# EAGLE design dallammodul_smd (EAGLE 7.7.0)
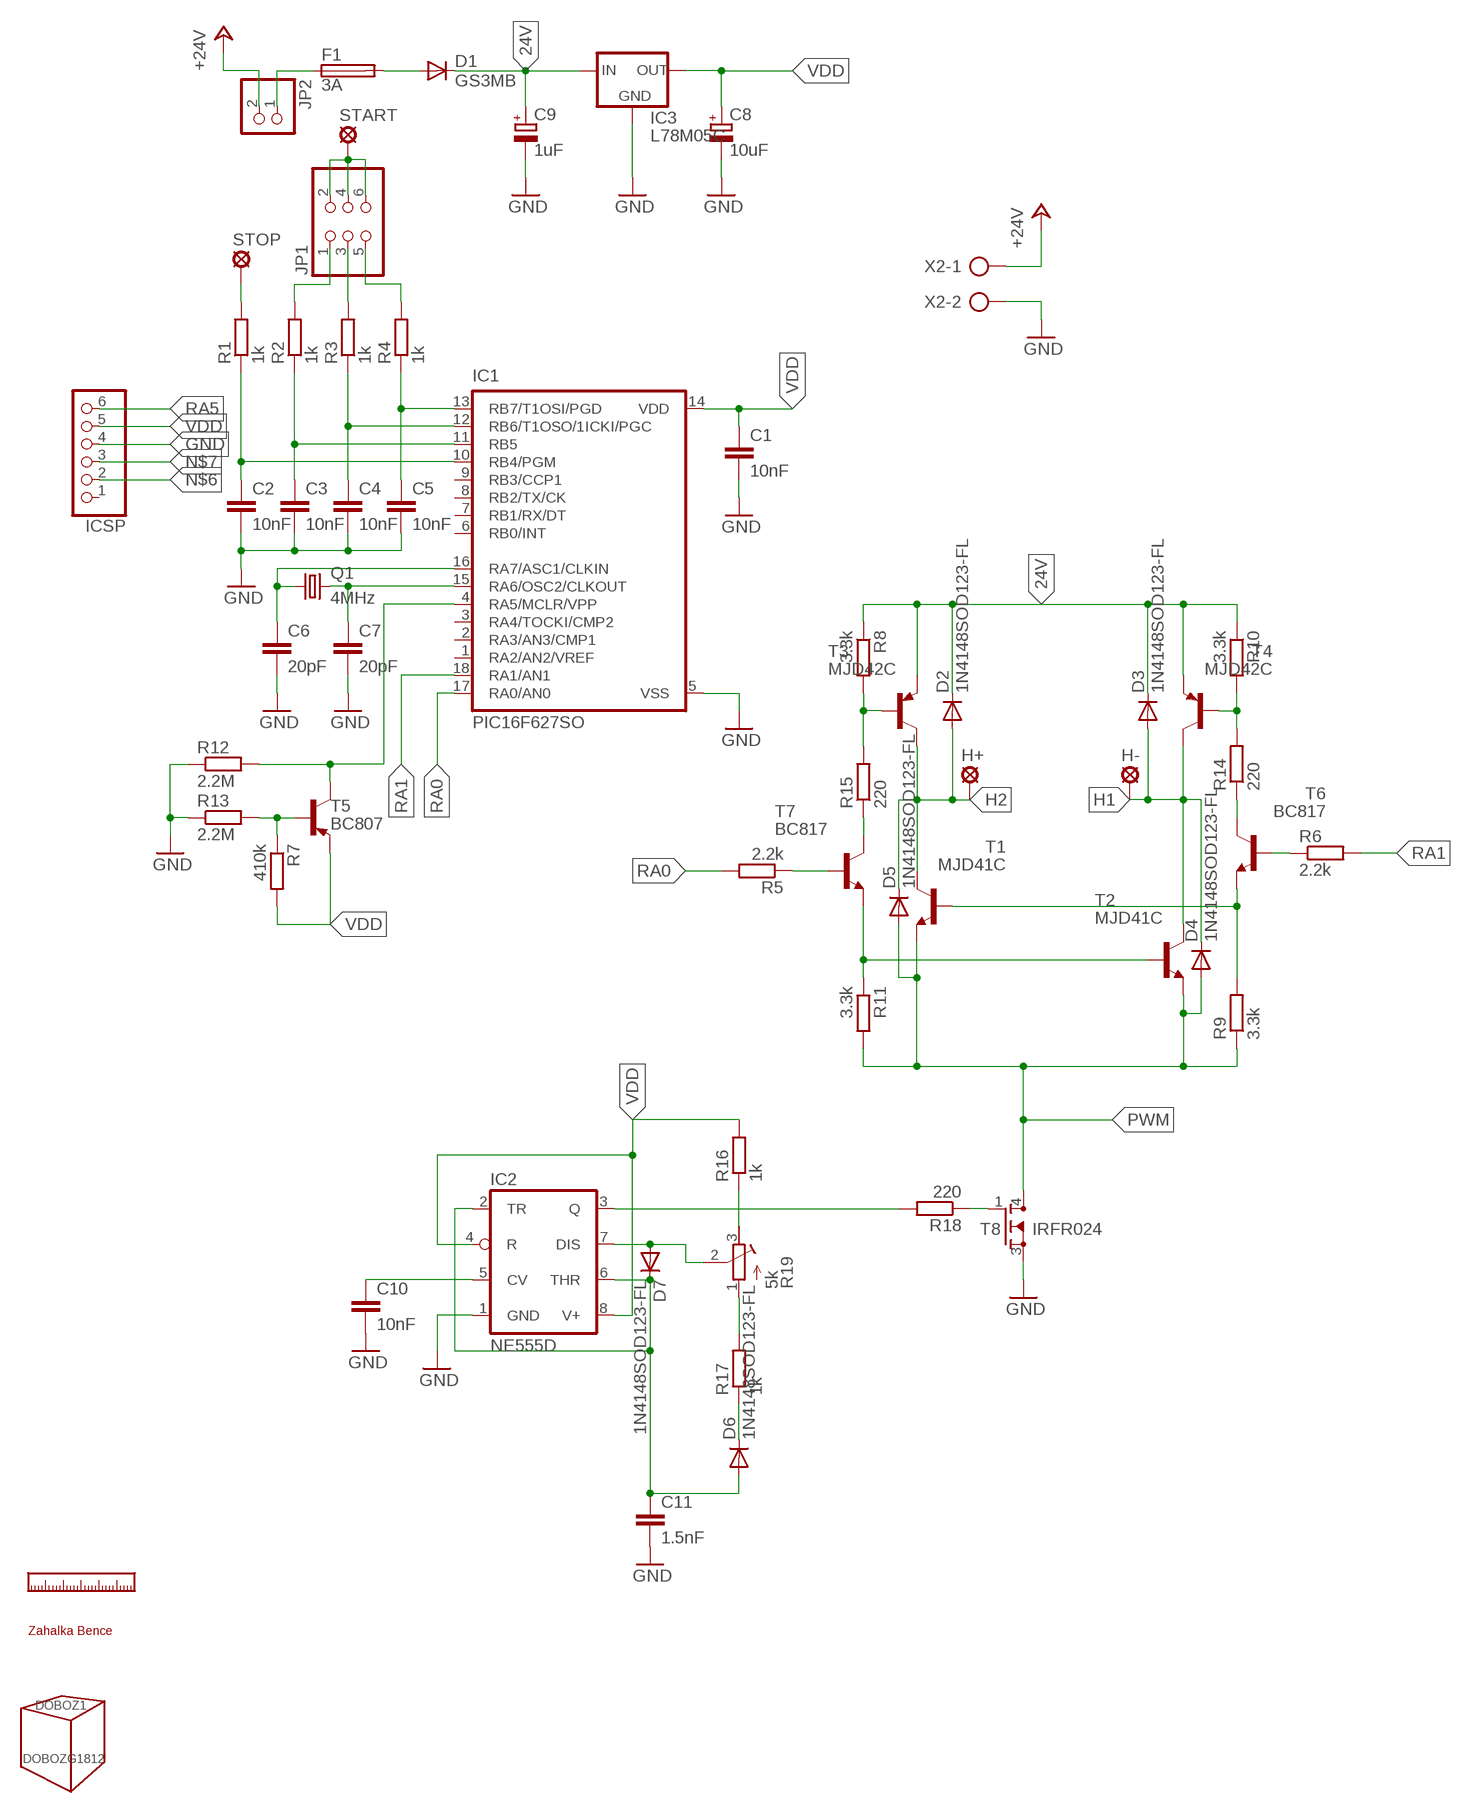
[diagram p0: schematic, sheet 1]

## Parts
C1  10nF  C-EUC0805  [C0805]
C2  10nF  C-EUC0805  [C0805]
C3  10nF  C-EUC0805  [C0805]
C4  10nF  C-EUC0805  [C0805]
C5  10nF  C-EUC0805  [C0805]
C6  20pF  C-EUC0805  [C0805]
C7  20pF  C-EUC0805  [C0805]
C8  10uF  CPOL-EU153CLV-0505  [153CLV-0505]
C9  1uF  CPOL-EU153CLV-0405  [153CLV-0405]
C10  10nF  C-EUC0805  [C0805]
C11  1.5nF  C-EUC0805  [C0805]
D1  GS3MB  DIODE-DO214AA  [DO214AA]
D2  1N4148SOD123-FL  [SOD123FL]
D3  1N4148SOD123-FL  [SOD123FL]
D4  1N4148SOD123-FL  [SOD123FL]
D5  1N4148SOD123-FL  [SOD123FL]
D6  1N4148SOD123-FL  [SOD123FL]
D7  1N4148SOD123-FL  [SOD123FL]
DOBOZ1  DOBOZG1812  [G1812]
F1  3A  BIZTOSITEK  [OMNIBLOK]
H+  LSP10  [LSP10]
H-  LSP10  [LSP10]
IC1  PIC16F627SO  [SO-18W]
IC2  NE555D  [SO08]
IC3  L78M05C  L78MXXCDPAK  [TO252]
ICSP  PINHD-1X6  [1X06]
JP1  PINHD-2X3  [2X03]
JP2  PINHD-1X2  [1X02]
Q1  4MHz  CRYSTALHC49UP  [HC49UP]
R1  1k  R-EU_R0805  [R0805]
R2  1k  R-EU_R0805  [R0805]
R3  1k  R-EU_R0805  [R0805]
R4  1k  R-EU_R0805  [R0805]
R5  2.2k  R-EU_R0805  [R0805]
R6  2.2k  R-EU_R0805  [R0805]
R7  410k  R-EU_R0805  [R0805]
R8  3.3k  R-EU_R0805  [R0805]
R9  3.3k  R-EU_R0805  [R0805]
R10  3.3k  R-EU_R0805  [R0805]
R11  3.3k  R-EU_R0805  [R0805]
R12  2.2M  R-EU_R0805  [R0805]
R13  2.2M  R-EU_R0805  [R0805]
R14  220  R-EU_R0805  [R0805]
R15  220  R-EU_R0805  [R0805]
R16  1k  R-EU_R0805  [R0805]
R17  1k  R-EU_R0805  [R0805]
R18  220  R-EU_R0805  [R0805]
R19  5k  R-TRIMM64W  [RTRIM64W]
START  LSP10  [LSP10]
STOP  LSP10  [LSP10]
T1  MJD41C  TRANSISTOR-NPNDPAK  [TO252]
T2  MJD41C  TRANSISTOR-NPNDPAK  [TO252]
T3  MJD42C  TRANSISTOR-PNPDPAK  [TO252]
T4  MJD42C  TRANSISTOR-PNPDPAK  [TO252]
T5  BC807  TRANSISTOR-PNPSOT23-BEC  [SOT23]
T6  BC817  TRANSISTOR-NPNSOT23-BEC  [SOT23]
T7  BC817  TRANSISTOR-NPNSOT23-BEC  [SOT23]
T8  IRFR024  NPN-FETDPAK  [TO252]
U$1  VONALZO  [VONALZO]
X2  AK300/2  [AK300/2]
ZB1  ZB  [ZB]

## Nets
24V: C9.+ D1.C D2.C D3.C IC3.1(IN) R8.1 R10.1 T3.3(E) T4.3(E)
+24V: JP2.2 X2.1
GND: C1.2 C2.2 C3.2 C4.2 C5.2 C6.2 C7.2 C8.- C9.- C10.2 C11.2 IC1.5(VSS) IC2.1(GND) IC3.4(GND) ICSP.4 R12.1 R13.1 T8.3(S) X2.2
H1: D3.A D4.C H-.MP T2.4(C) T4.4(C)
H2: D2.A D5.C H+.MP T1.4(C) T3.4(C)
N$1: C6.1 IC1.16(RA7/ASC1/CLKIN) Q1.1
N$2: C7.1 IC1.15(RA6/OSC2/CLKOUT) Q1.2
N$3: C2.1 IC1.10(RB4/PGM) R1.1
N$4: C3.1 IC1.11(RB5) R2.1
N$5: R5.1 T7.1(B)
N$6: C4.1 IC1.12(RB6/T1OSO/1ICKI/PGC) ICSP.2 R3.1
N$7: C5.1 IC1.13(RB7/T1OSI/PGD) ICSP.3 R4.1
N$8: JP1.5 R4.2
N$9: JP1.3 R3.2
N$10: JP1.1 R2.2
N$11: R1.2 STOP.MP
N$12: R16.1 R19.3(A)
N$13: R17.2 R19.1(E)
N$14: D1.A F1.2
N$15: R8.2 R15.2 T3.1(B)
N$16: R10.2 R14.2 T4.1(B)
N$17: R7.1 R13.2 T5.1(B)
N$18: R15.1 T7.3(C)
N$19: R6.1 T6.1(B)
N$20: R11.1 T2.1(B) T7.2(E)
N$21: IC2.3(Q) R18.2
N$22: R9.2 T1.1(B) T6.2(E)
N$23: R14.1 T6.3(C)
N$24: R18.1 T8.1(G)
N$25: JP1.2 JP1.4 JP1.6 START.MP
N$26: D7.A IC2.7(DIS) R19.2(S)
N$27: D6.C R17.1
N$28: C11.1 D6.A D7.C IC2.2(TR) IC2.6(THR)
N$30: C10.1 IC2.5(CV)
N$31: F1.1 JP2.1
PWM: D4.A D5.A R9.1 R11.2 T1.3(E) T2.3(E) T8.4(D)
RA0: IC1.17(RA0/AN0) R5.2
RA1: IC1.18(RA1/AN1) R6.2
RA5: IC1.4(RA5/MCLR/VPP) ICSP.6 R12.2 T5.3(C)
VDD: C1.1 C8.+ IC1.14(VDD) IC2.4(R) IC2.8(V+) IC3.3(OUT) ICSP.5 R7.2 R16.2 T5.2(E)
Unconnected: IC1.1(RA2/AN2/VREF) IC1.2(RA3/AN3/CMP1) IC1.3(RA4/TOCKI/CMP2) IC1.6(RB0/INT) IC1.7(RB1/RX/DT) IC1.8(RB2/TX/CK) IC1.9(RB3/CCP1) ICSP.1

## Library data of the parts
C1-C7 C10 C11 = rcl:C-EU: CAPACITOR, European symbol
C8 C9 = rcl:CPOL-EU: POLARIZED CAPACITOR, European symbol
D1 = diode:DIODE-: DIODE
D2-D7 = diode:1N4148: DIODE
DOBOZ1 = sajat:DOBOZ: Ha eleve dobozba tervezném az áramkört, akkor miért ne legyen meg alkatrészként?
F1 = sajat:BIZTOSITEK
H+ H- START STOP = sajat:LSP10: SOLDER PAD
IC1 = microchip:PIC16*F62: FLASH-Based 8-Bit CMOS Microcontroller Source: http://ww1.microchip.com/downloads/en/DeviceDoc/40300C.pdf; MF: MICROCHIP; MPN: PIC16F627-04/SO; OC_FARNELL: 1084265; OC_NEWARK: 69K7632
IC2 = linear:*555: TIMER
IC3 = sajat:L78MXXC
ICSP = pinhead:PINHD-1X6: PIN HEADER
JP1 = pinhead:PINHD-2X3: PIN HEADER
JP2 = pinhead:PINHD-1X2: PIN HEADER
Q1 = crystal:CRYSTAL: CRYSTAL; OC_FARNELL: unknown; OC_NEWARK: unknown
R1-R18 = rcl:R-EU_: RESISTOR, European symbol
R19 = resistor:R-TRIMM: Trimm resistor
T1 T2 T6 T7 = sajat:TRANSISTOR-NPN
T3-T5 = sajat:TRANSISTOR-PNP
T8 = sajat:NPN-FET: NPN FET
U$1 = sajat:VONALZO: vonalzó
X2 = con-ptr500:AK300/2: CONNECTOR; OC_FARNELL: unknown; OC_NEWARK: unknown
ZB1 = sajat:ZB: Zahalka Bence monogram

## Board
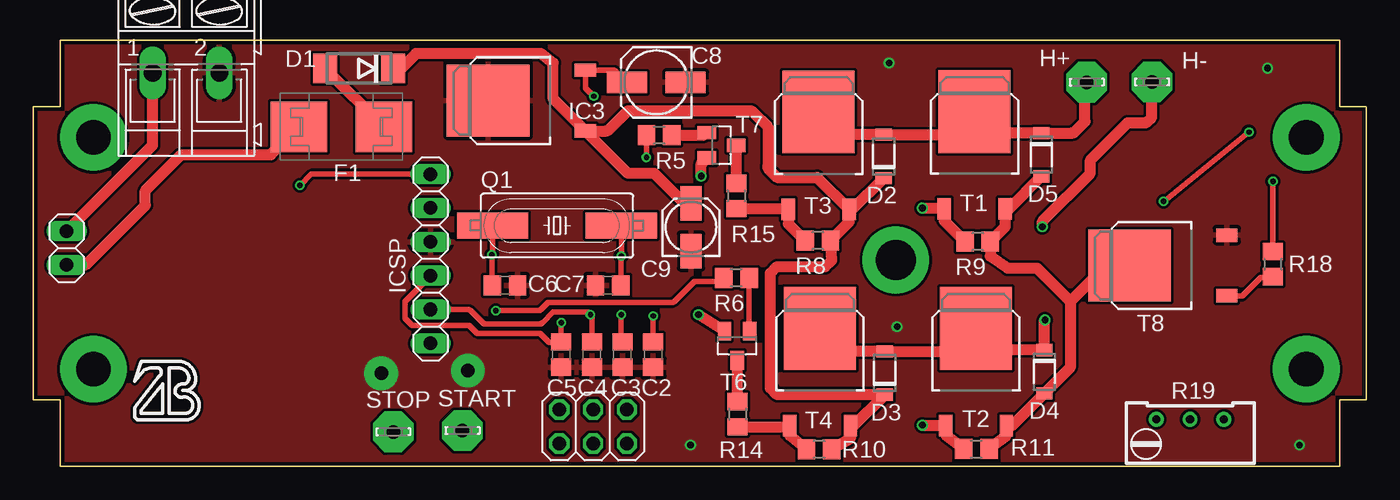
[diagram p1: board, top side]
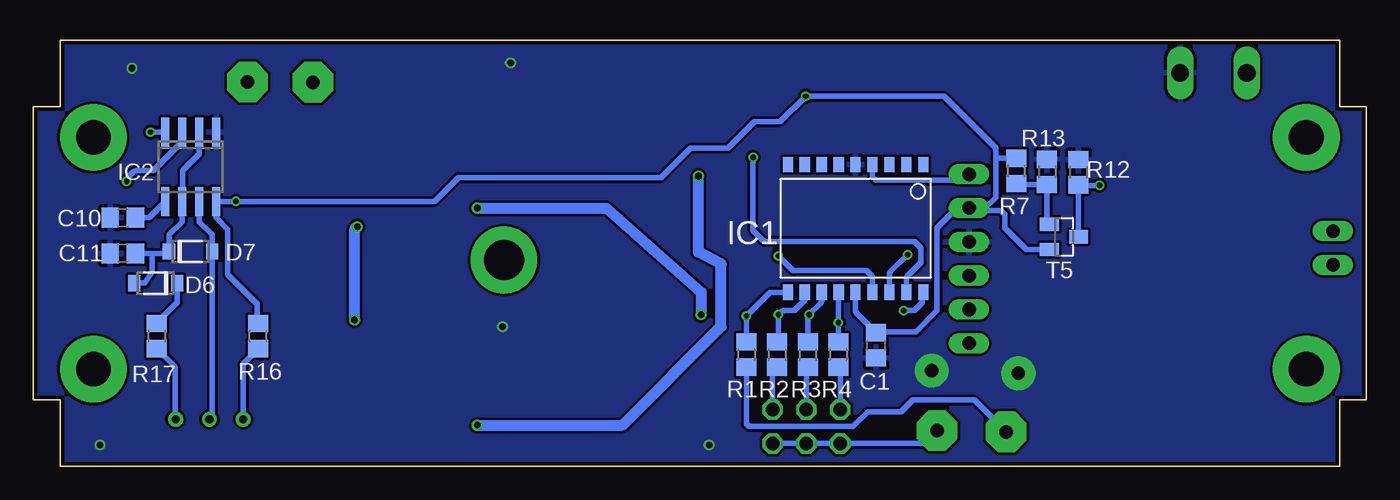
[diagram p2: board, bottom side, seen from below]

Size 100 x 32 mm. Coordinates in mm from the lower left corner, seen from the top.
Copper layers (1*16): Top 0.035mm / dielectric 1.5mm / Bottom 0.035mm
Design rules "dirt_cheap_dirty_boards.v1": minimum track width 5mil, minimum drill 12mil, track to track 5mil, track to pad 5mil, pad to pad 5mil, via to via 5mil, smd to smd 0mil, copper to edge 10mil, drill to drill 10mil, minimum pad ring 10mil, minimum via ring 6mil, stop-mask expansion 2mil, vias tented up to drill 25mil, thermal gap 10mil

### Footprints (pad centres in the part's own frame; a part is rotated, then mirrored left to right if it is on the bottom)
C0805 = smd 1.3 x 1.5: 1 -0.95,0; 2 0.95,0
153CLV-0505 = smd 3 x 1.6: + 2.2,0; - -2.2,0
153CLV-0405 = smd 2.6 x 1.6: + 1.8,0; - -1.8,0
DO214AA = smd 1.8 x 2.2: A 2.55,0; C -2.55,0
SOD123FL = smd 0.91 x 1.22: A 1.625,0; C -1.625,0
G1812 = drill 2.6 pad 5: P$1 -45.5,-8.7; P$2 45.5,-8.7; P$3 45.5,8.7; P$4 -45.5,8.7
OMNIBLOK = smd 4.24 x 3.81: 1 -3.185,0; 2 3.185,0
LSP10 = drill 1.016 pad 3.048 octagon: MP 0,0
SO-18W = smd 0.762 x 1.143: 1 -5.08,-4.788; 2 -3.81,-4.788; 3 -2.54,-4.788; 4 -1.27,-4.788; 5 0,-4.788; 6 1.27,-4.788; 7 2.54,-4.788; 8 3.81,-4.788; 9 5.08,-4.788; 10 5.08,4.788; 11 3.81,4.788; 12 2.54,4.788; 13 1.27,4.788; 14 0,4.788; 15 -1.27,4.788; 16 -2.54,4.788; 17 -3.81,4.788; 18 -5.08,4.788
SO08 = smd 0.6 x 2.2: 1 -1.905,-2.6; 2 -0.635,-2.6; 3 0.635,-2.6; 4 1.905,-2.6; 5 1.905,2.6; 6 0.635,2.6; 7 -0.635,2.6; 8 -1.905,2.6
TO252 = smd 1 x 1.6: 1 -2.28,-4.8; 3 2.28,-4.8 | smd 5.4 x 6.2: 4 0,2.5
1X06 = drill 1.016 long: 1 -6.35,0; 2 -3.81,0; 3 -1.27,0; 4 1.27,0; 5 3.81,0; 6 6.35,0
2X03 = drill 1.016 octagon: 1 -2.54,-1.27; 2 -2.54,1.27; 3 0,-1.27; 4 0,1.27; 5 2.54,-1.27; 6 2.54,1.27
1X02 = drill 1.016 long: 1 -1.27,0; 2 1.27,0
HC49UP = smd 5.334 x 1.93: 1 -4.826,0; 2 4.826,0
R0805 = smd 1.3 x 1.5: 1 -0.95,0; 2 0.95,0
RTRIM64W = drill 0.61: 1 1.27,-2.54; 2 1.27,0; 3 1.27,2.54
SOT23 = smd 1 x 1.4: 1 -0.95,-1.1; 2 0.95,-1.1; 3 0,1.1
AK300/2 = drill 1.321 long: 1 -2.515,0; 2 2.489,0

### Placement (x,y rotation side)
C1  36.78,9.1 270 bottom
C2  46.5,8.4 270 top
C3  44.2,8.4 270 top
C4  41.9,8.4 270 top
C5  39.6,8.4 270 top
C6  35.38,13.6 0 top
C7  43.13,13.6 180 top
C8  46.74,28.84 180 top
C9  49.34,17.97 90 top
C10  93.28,18.68 180 bottom
C11  93.28,16 180 bottom
D1  24.46,29.88 180 top
D2  63.8,23.28 90 top
D3  63.88,7.02 90 top
D4  75.85,7.11 270 top
D5  75.63,23.41 270 top
D6  90.82,13.76 180 bottom
D7  88.2,16.14 0 bottom
DOBOZ1  50,16 0 top
F1  23.1,25.5 0 top
H+  79.03,28.85 0 top
H-  83.93,28.87 0 top
IC1  38.31,17.87 180 bottom
IC2  88.2,22.49 180 bottom
IC3  36.62,27.47 90 top
ICSP  29.8,15.6 90 top
JP1  42,3 180 top
JP2  2.5,16.4 90 top
Q1  39.29,18.09 0 top
R1  46.5,8.4 270 bottom
R2  44.2,8.4 270 bottom
R3  41.9,8.4 270 bottom
R4  39.6,8.4 270 bottom
R5  46.95,24.86 180 top
R6  52.75,14.16 180 top
R7  26.24,22.19 90 bottom
R8  58.85,16.96 180 top
R9  70.85,16.88 180 top
R10  58.95,1.28 180 top
R11  70.75,1.32 0 top
R12  21.59,22.09 270 bottom
R13  23.94,22.11 270 bottom
R14  52.84,3.93 270 top
R15  52.74,20.31 270 top
R16  83.12,9.79 90 bottom
R17  90.74,9.79 270 bottom
R18  93.01,15.19 90 top
R19  86.79,2.27 90 top
START  32.2,2.7 0 top
STOP  27,2.6 0 top
T1  70.62,24.14 0 top
T2  70.72,7.86 0 top
T3  58.92,24.11 0 top
T4  59.02,7.86 0 top
T5  22.67,17.24 270 bottom
T6  52.8,9.07 180 top
T7  51.63,24.12 270 top
T8  84.74,15.09 90 top
U$1  not placed on the board
X2  11.47,29.55 0 top
ZB1  9.9,5.8 0 top

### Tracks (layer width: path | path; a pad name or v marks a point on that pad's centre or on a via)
24V
  Top 0.813: T3.3 61.2,18.36 R8.1 59.9,15.5 59.4,15 55.8,15 55.3,14.5 55.3,5.9 55.8,5.39 D3.C 61.55,3.06 T4.3 61.3,2.08 R10.1 | T3.3 61.45,19.31 D2.C | T3.3 58.81,21.7 55.8,21.7 55.19,22.31 arc-45 55.1,22.53 55.1,25.5 53.99,26.61 arc45 53.77,26.7 44.6,26.7 43.18,25.28 arc-45 42.96,25.19 IC3.1 | C9.+ 48.96,19.77 arc-45 48.74,19.86 46.6,22 44.74,22 arc-45 44.52,22.09 IC3.1 | IC3.1 39,27.6 39,30.28 38.08,31 28.7,31 27.58,29.88 D1.C
+24V
  Top 0.813: JP2.2 8.96,24.13 X2.1
GND  (via drill 0.5, 1 pad 2.54)
  other vias: 64.2,30.3 92.6,29.9 95,1.6 49.3,1.6 32.6,7.2 26.1,7 64.8,10.5
  pour Bottom (isolate 0.2): 2,32 98,32 98,27 100,27 100,5 98,5 98,0 2,0 2,5 0,5 0,27 2,27
  pour Top (isolate 0.2): 0,32.2 100.1,32.2 100.1,-1.3 0,-1.3 0,30.2
H1  (via drill 0.5)
  Top 0.813: T4.4 60.73,8.64 D3.A 69,8.64 T2.4 72.34,8.73 D4.C 75.85,10.88 arc-45 v75.9,11 | v75.7,18 75.7,18.27 arc-45 75.79,18.49 79.3,22 79.3,22.87 arc-45 79.39,23.09 82.1,25.8 83.37,25.8 arc45 83.59,25.89 83.9,26.2 83.9,28.8 arc-45 H-.MP
  Bottom 0.813: v75.9,11 75.9,17.67 arc45 75.81,17.89 v75.7,18
H2
  Top 0.813: 70.98,26.28 72.22,25.04 D5.C 77.9,25.04 arc45 78.13,25.13 78.9,25.9 78.9,28.59 arc-45 78.99,28.81 H+.MP | 70.98,26.28 T1.4 | T3.4 60.62,24.9 D2.A 69.61,24.9 70.98,26.28
HUTOBORDA  (via drill 3 pad 5)
  other vias: 64.7,15.5
N$1  (via drill 0.4)
  Top 0.406: Q1.1 34.46,16.05 arc-45 v34.4,15.9 arc-45 34.43,15.83 C6.1
  Bottom 0.406: IC1.16 35.77,14.4 arc45 35.68,14.62 v34.4,15.9
N$2  (via drill 0.4)
  Top 0.406: Q1.2 44.12,15.84 arc-45 v44.1,15.8 arc45 44.08,15.75 C7.1
  Bottom 0.406: IC1.15 37.04,14.11 arc-45 37.13,14.33 37.5,14.7 42.87,14.7 arc45 43.09,14.79 v44.1,15.8
N$3  (via drill 0.4)
  Top 0.406: v46.5,11.3 C2.1
  Bottom 0.406: C2.1 v46.5,11.3 44.81,12.99 arc45 44.59,13.08 IC1.10
N$4  (via drill 0.4)
  Top 0.406: v44.1,11.4 44.1,9.58 arc45 C3.1
  Bottom 0.406: C3.1 C3.1 arc-45 44.1,9.58 v44.1,11.4 43.89,11.61 arc45 43.67,11.7 42.9,11.7 42.21,12.39 arc-45 42.12,12.61 IC1.11
N$5
  Top 0.813: R5.1 50.19,24.86 arc45 50.41,24.95 T7.1
N$6  (via drill 0.4)
  Top 0.406: C4.1 41.9,11.17 arc45 v41.81,11.39 v41.8,11.4 41.6,11.6 39,11.6 38.19,10.79 arc-45 37.97,10.7 33.8,10.7 32.8,11.7 arc45 32.58,11.79 ICSP.2
  Bottom 0.406: C4.1 41.9,11.3 arc90 v41.8,11.4 40.94,12.26 arc-45 40.85,12.48 IC1.12
N$7  (via drill 0.4)
  Top 0.406: v39.6,10.8 C5.1 39.55,9.3 38.7,9.3 38,10 33.3,10 32.7,10.6 28.4,10.6 27.9,11.1 27.9,12.4 29.8,14.3 ICSP.3
  Bottom 0.406: C5.1 v39.6,10.8 arc-45 39.58,10.85 IC1.13
N$8
  Bottom 0.406: JP1.5 39.46,7.18 arc-45 39.55,7.4 R4.2
N$9
  Bottom 0.406: JP1.3 42,7.22 arc45 R3.2
N$10
  Bottom 0.406: JP1.1 44.54,6.98 arc45 44.45,7.2 R2.2
N$11
  Bottom 0.406: R1.2 46.5,3.2 46.3,3 38.5,3 37.4,4.1 34.9,4.1 34,5 29.4,5 STOP.MP
N$12
  Bottom 0.406: R16.1 84.18,7.78 arc-45 84.27,7.56 84.27,3.56 R19.3
N$13
  Bottom 0.406: R17.2 89.44,7.54 arc45 89.35,7.32 89.35,3.56 R19.1
N$14
  Top 0.813: D1.A F1.2
N$15
  Top 0.813: R8.2 56.64,18.22 T3.1 56.59,19.36 R15.2
N$16
  Top 0.813: R10.2 56.74,2.34 T4.1 56.66,2.98 R14.2
N$17
  Bottom 0.406: T5.1 23.94,18.36 R13.2 26.16,21.16 R7.1
N$18
  Top 0.813: T7.3 52.72,21.28 R15.1
N$19
  Top 0.406: R6.1 53.7,10.22
  Top 0.813: 53.7,10.22 T6.1
N$20  (via drill 0.5 pad 0.81)
  Top 0.813: R11.1 68.44,2.38 T2.1 68.4,3.1 v66.7,3.1 | v50.1,21.8 50.1,22.61 arc-45 50.19,22.83 T7.2
  Bottom 0.813: v66.7,3.1 55.8,3.1 48.4,10.5 48.4,15.2 50.1,16.1 v50.1,21.8
N$21  (via drill 0.4)
  Top 0.406: v93,21.4 93,16.2 R18.2
  Bottom 0.406: IC2.3 88.83,24.5 arc45 88.93,24.27 91,22.2 92.27,22.2 arc-45 92.49,22.11 92.9,21.7 92.9,21.5 v93,21.4
N$22  (via drill 0.5 pad 0.81)
  Top 0.813: R9.2 68.34,18.44 T1.1 68.28,19.4 v66.7,19.4 | v49.9,11.4 51.82,10.2 T6.2
  Bottom 0.813: v66.7,19.4 57,19.4 49.9,13.1 v49.9,11.4
N$23
  Top 0.813: T6.3 52.8,4.92 R14.1
N$24
  Top 0.406: R18.1 93,14.2 92.1,14.2 90.7,12.8 89.6,12.8 T8.1
N$25
  Bottom 0.406: JP1.2 JP1.4 JP1.6 33.17,1.73 START.MP
N$26
  Bottom 0.406: IC2.7 87.56,18.37 86.6,17.4 86.6,16.16 D7.A 86.58,3.75 R19.2
N$27
  Bottom 0.406: D6.C 89.2,13.7 89.2,12.3 90.7,10.8 R17.1
N$28
  Bottom 0.406: IC2.2 87.56,23.43 88.8,22.2 88.8,19.93 IC2.6 88.83,18.37 89.8,17.4 89.8,16.16 D7.C 89.97,16 91.1,16 | C11.1 91.1,16 | D6.A 91.64,13.76 91.1,14.6 91.1,16
N$30
  Bottom 0.406: C10.1 91.31,18.68 IC2.5
N$31
  Top 0.813: JP2.1 3.93,15.13 8.4,19.6 8.4,20.7 11.1,23.4 17.82,23.4 F1.1
PWM
  Top 0.813: R11.2 73,2.32 T2.3 73.42,3.06 D4.A 77.8,7.44 77.8,12.4 | D5.A 73.19,19.34 T1.3 72.9,17.98 R9.1 71.8,15.8 73.1,14.9 75.3,14.9 77.8,12.4 | T8.4 80.26,14.96 arc-45 80.19,14.79 77.8,12.4
RA0  (via drill 0.4)
  Top 0.406: R5.2 v46,23.2
  Bottom 0.406: IC1.17 34.5,14.07 arc45 34.41,14.29 33.4,15.3 33.4,16.27 arc-45 33.49,16.49 33.9,16.9 45.07,16.9 arc45 45.29,16.99 46,17.7 v46,23.2
RA1  (via drill 0.4)
  Top 0.406: v34.7,11.7 37.87,11.7 arc45 38.09,11.79 38.6,12.3 47.87,12.3 arc45 48.09,12.39 49.6,13.9 51.41,13.9 arc45 51.63,13.99 R6.2
  Bottom 0.406: v34.7,11.7 34.03,11.7 arc-45 33.81,11.79 33.3,12.3 33.3,12.91 arc45 IC1.18
RA5  (via drill 0.4)
  Top 0.406: ICSP.6 20.85,21.95 v20,21.1
  Bottom 0.406: IC1.4 37.04,21.74 36.8,21.5 30.25,21.5 ICSP.6 | T5.3 21.59,17.26 R12.2 21.55,21.1 v20,21.1
VDD  (via drill 0.4)
  Top 0.406: v84.8,19.9 v91.2,25.1 | C8.+ 43.72,29.66 arc45 43.5,29.75 IC3.3 41.42,28.42 v42.04,27.8
  Bottom 0.406: R16.2 83.2,10.82 83.2,12.2 85.4,14.4 85.4,17.8 86.3,18.7 IC2.8 v84.8,19.9 69.9,19.9 68.1,21.7 52.9,21.7 50.7,23.9 47.9,23.9 45.9,25.9 44,25.9 v42.04,27.8 31.7,27.8 27.8,23.9 27.8,23.1 | v91.2,25.1 IC2.4 | IC1.14 38.31,11.71 arc-45 38.22,11.49 C1.1 36.73,10.1 33.8,10.1 32.2,11.7 32.2,17.9 30.69,19.41 ICSP.5 28.9,19.4 | 27.8,23.1 27.8,20.2 28.6,19.4 28.9,19.4 | T5.2 25.49,16.29 27.1,17.9 27.1,18.9 27.4,19.2 28.7,19.2 28.9,19.4 | R7.2 27.76,23.14 27.8,23.1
